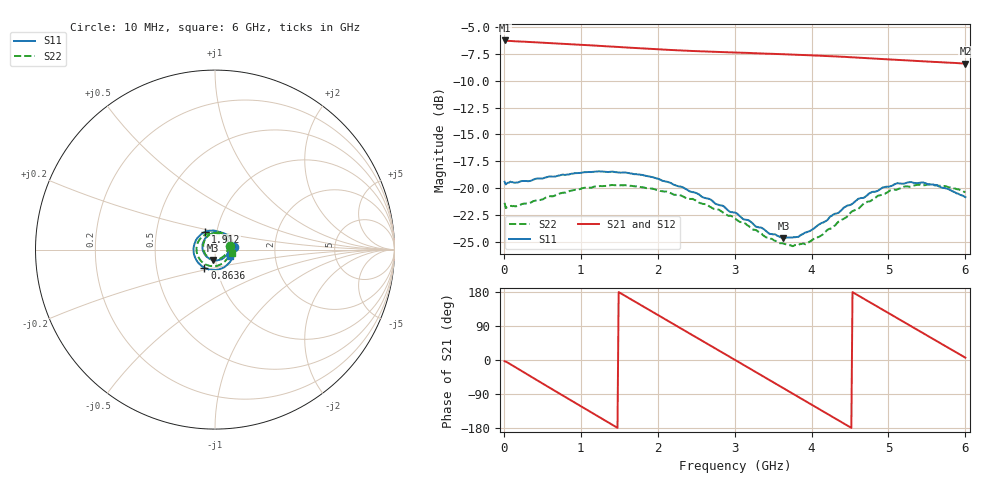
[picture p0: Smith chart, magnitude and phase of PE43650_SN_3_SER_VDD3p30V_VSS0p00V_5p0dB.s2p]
!Keysight Technologies,N5245B,MY57181451,A.13.50.07
!Date: Tuesday, May 07, 2019 07:59:54
!Correction: S11(Full 2 Port(1,2))
!S21(Full 2 Port(1,2))
!S12(Full 2 Port(1,2))
!S22(Full 2 Port(1,2))
!S2P File: Measurements: S11, S21, S12, S22:
# Hz S  dB  R 50
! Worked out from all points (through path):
!   401 points, 10 MHz to 6 GHz, reference 50 ohm
!   highest |S21| = -6.28 dB at 10 MHz (marker M1); lowest = -8.4 dB at 6 GHz (marker M2)
!   group delay of S21, straight-line fit = 330 ps
!   lowest |S11| = -24.6 dB at 3.634 GHz (marker M3), VSWR 1.12, Z = 48.7 - j5.66 ohm
!   |S11| at or under -10 dB: start of sweep to end of sweep
!   |S22| runs from -25.4 to -19.6 dB; largest |S21 - S12| = 0.0035
!   S11 on the Smith chart (normalised r, x): 10 MHz: 1.24, +0.04; 863.6 MHz: 0.87, -0.18; 1.912 GHz: 0.88, +0.18; 6 GHz: 1.18, -0.08
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1e7  -19.38 8.7  -6.28 -3.2  -6.33 -3.4  -21.33 13.6
2.34625e8  -19.32 -34.9  -6.39 -29.4  -6.44 -29.3  -21.45 -35.0
4.892e8  -19.08 -70.7  -6.48 -60.3  -6.53 -60.3  -21.03 -71.3
8.63575e8  -18.67 -120.6  -6.62 -105.5  -6.67 -105.6  -20.22 -120.4
1.013325e9  -18.55 -139.3  -6.69 -123.6  -6.74 -123.6  -19.99 -138.4
1.462575e9  -18.50 168.4  -6.87 -177.3  -6.94 -177.2  -19.70 171.8
1.911825e9  -18.92 119.3  -7.06 129.4  -7.12 129.4  -20.00 125.8
2.01665e9  -19.13 108.4  -7.11 116.9  -7.16 117.0  -20.19 115.5
2.241275e9  -19.74 84.4  -7.19 90.4  -7.24 90.4  -20.60 93.1
2.4659e9  -20.35 59.7  -7.26 63.9  -7.31 63.9  -21.02 70.5
2.750425e9  -21.42 28.2  -7.34 30.3  -7.39 30.4  -21.93 40.3
3.005e9  -22.24 -3.9  -7.40 0.2  -7.46 0.3  -22.76 11.3
3.289525e9  -23.56 -43.6  -7.47 -33.5  -7.52 -33.4  -23.90 -27.2
3.63395e9  -24.62 -99.6  -7.56 -74.3  -7.61 -74.2  -25.11 -80.4
4.008325e9  -23.82 -163.6  -7.66 -118.7  -7.71 -118.7  -24.78 -145.0
4.2629e9  -22.53 158.1  -7.74 -148.9  -7.80 -148.8  -23.68 174.8
4.5025e9  -21.54 125.8  -7.83 -177.4  -7.89 -177.2  -22.31 140.7
4.7421e9  -20.50 96.4  -7.93 154.2  -7.98 154.4  -21.21 111.8
5.01165e9  -19.82 67.0  -8.04 122.5  -8.09 122.6  -20.22 81.0
5.4609e9  -19.47 22.7  -8.22 69.5  -8.26 69.7  -19.70 36.4
5.745425e9  -20.00 -2.0  -8.33 36.0  -8.37 36.1  -19.79 10.6
6e9  -20.81 -21.6  -8.42 6.1  -8.47 6.2  -20.36 -10.6
